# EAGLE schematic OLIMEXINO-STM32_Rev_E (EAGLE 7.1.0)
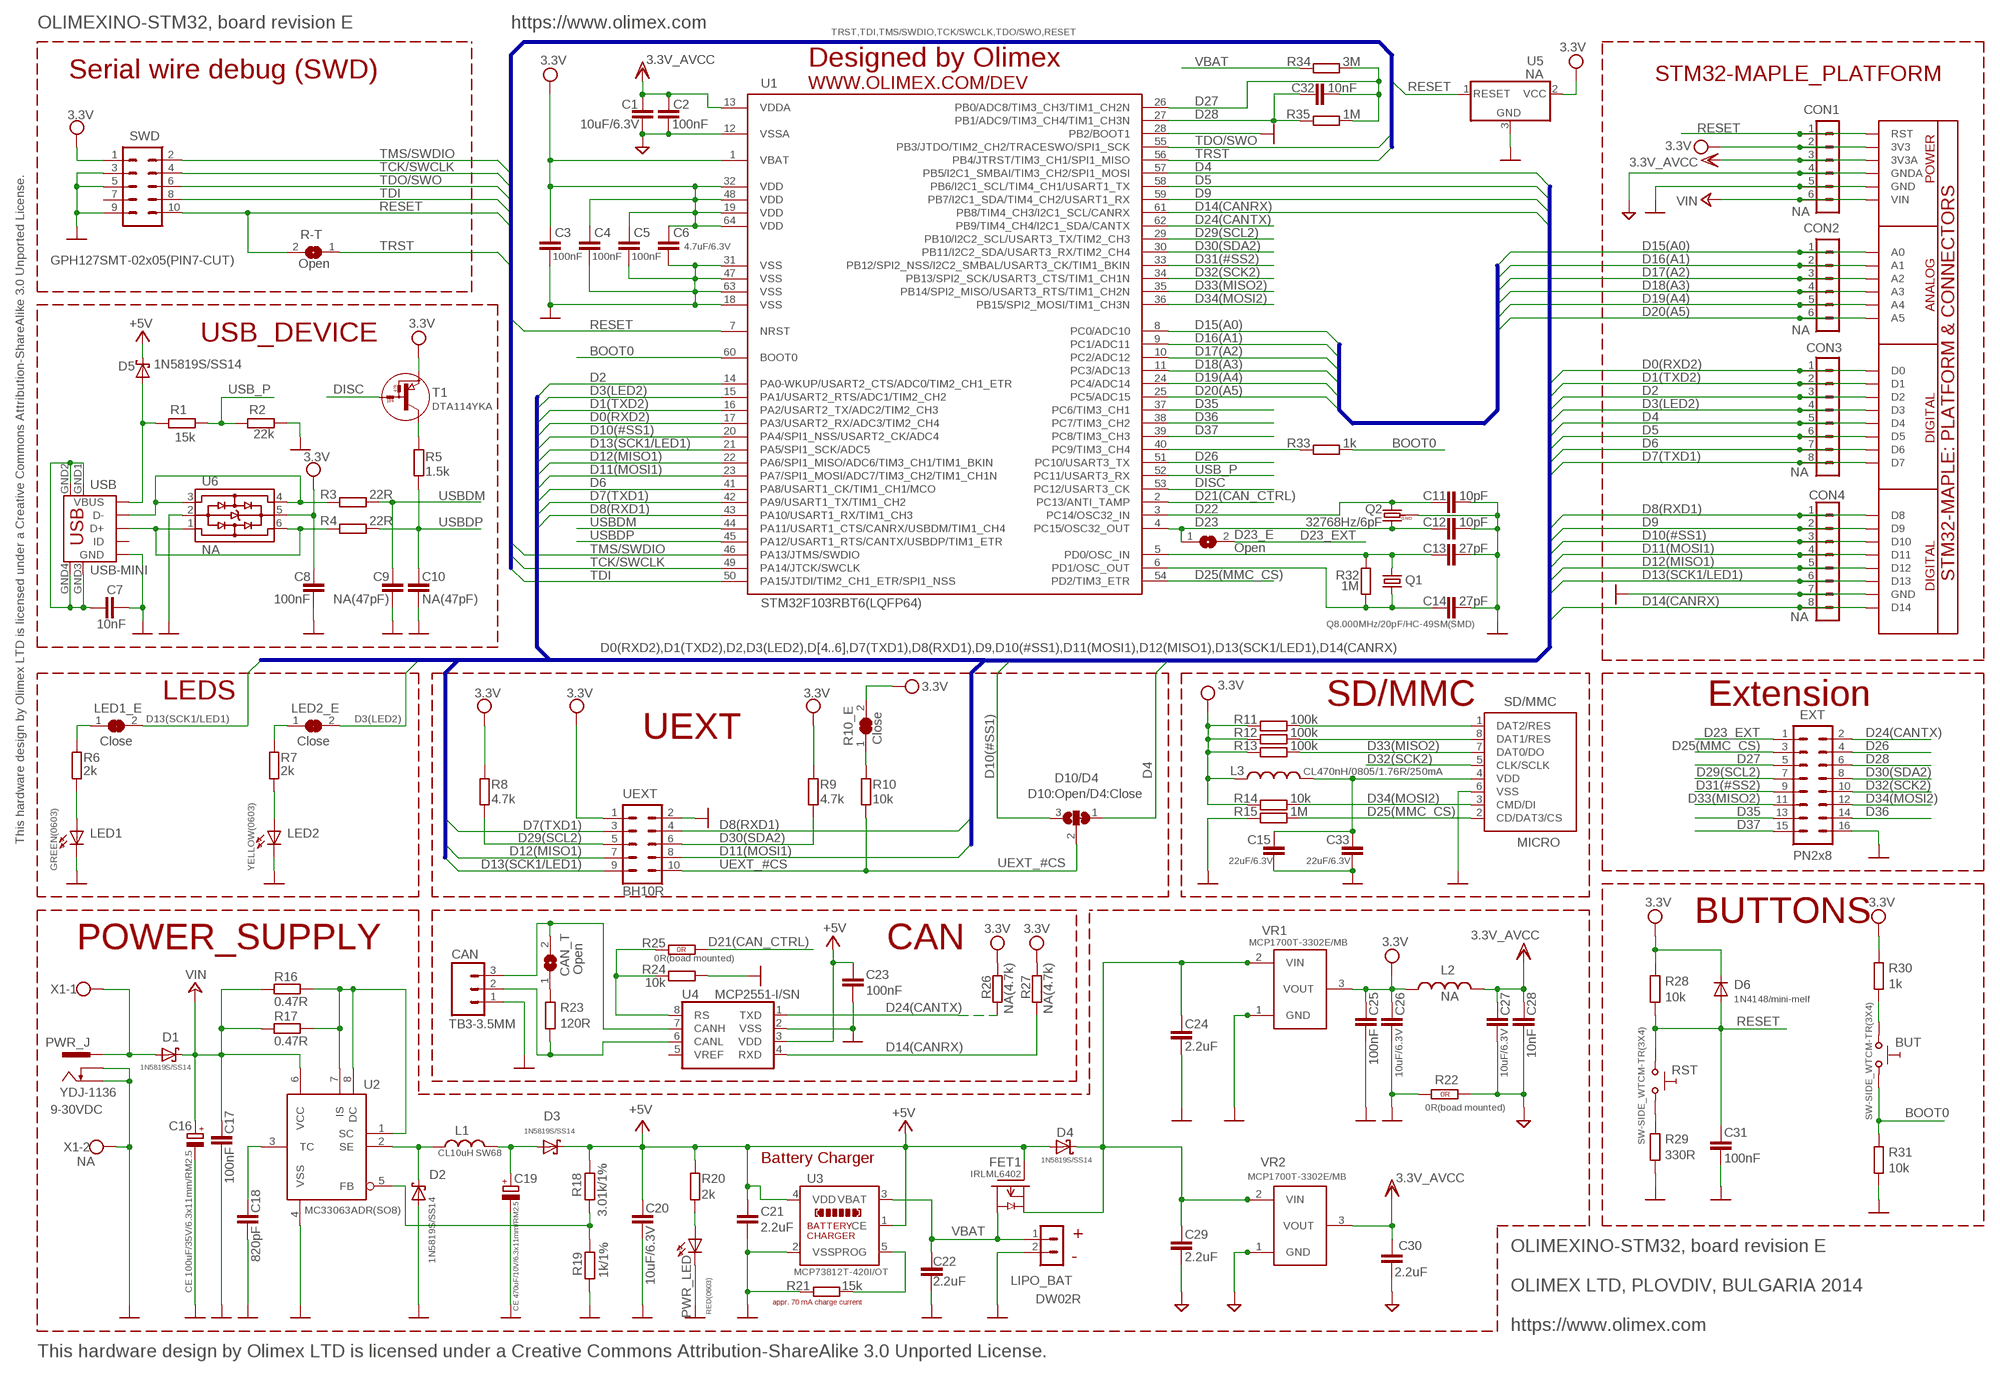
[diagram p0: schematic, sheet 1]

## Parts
BUT  SW-SIDE_WTCM-TR(3X4)  SW-TAKTSIDE_WTCM-TR(3X4)  [SW_TAKT3X4]
C1  10uF/6.3V  C-EUC0805_5MIL_DWS  [C0805_5MIL_DWS]
C2  100nF  C-EUC0603_DWS  [C0603_DWS]
C3  100nF  C-EUC0603_DWS  [C0603_DWS]
C4  100nF  C-EUC0603_DWS  [C0603_DWS]
C5  100nF  C-EUC0603_DWS  [C0603_DWS]
C6  4.7uF/6.3V  C-EUC0603_DWS  [C0603_DWS]
C7  10nF  C-EUC0603_DWS  [C0603_DWS]
C8  100nF  C-EUC0603_DWS  [C0603_DWS]
C9  NA(47pF)  C-EUC0603_DWS_NA  [C0603_DWS_NA]
C10  NA(47pF)  C-EUC0603_DWS_NA  [C0603_DWS_NA]
C11  10pF  C-EUC0603_DWS  [C0603_DWS]
C12  10pF  C-EUC0603_DWS  [C0603_DWS]
C13  27pF  C-EUC0603_DWS  [C0603_DWS]
C14  27pF  C-EUC0603_DWS  [C0603_DWS]
C15  22uF/6.3V  C-EUC0603_DWS  [C0603_DWS]
C16  CE 100uF/35V/6.3x11mm/RM2.5  CPOL-EUE2.5-6.3  [E2,5-6,3]
C17  100nF  C-EUC0603_DWS  [C0603_DWS]
C18  820pF  C-EUC0603_DWS  [C0603_DWS]
C19  CE 470uF/10V/6.3x11mm/RM2.5  CPOL-EUE2.5-6.3  [E2,5-6,3]
C20  10uF/6.3V  C-EUC0805_5MIL_DWS  [C0805_5MIL_DWS]
C21  2.2uF  C-EUC0603_DWS  [C0603_DWS]
C22  2.2uF  C-EUC0603_DWS  [C0603_DWS]
C23  100nF  C-EUC0603_DWS  [C0603_DWS]
C24  2.2uF  C-EUC0603_DWS  [C0603_DWS]
C25  100nF  C-EUC0603_DWS  [C0603_DWS]
C26  10uF/6.3V  C-EUC0805_5MIL_DWS  [C0805_5MIL_DWS]
C27  10uF/6.3V  C-EUC0805_5MIL_DWS  [C0805_5MIL_DWS]
C28  10nF  C-EUC0603_DWS  [C0603_DWS]
C29  2.2uF  C-EUC0603_DWS  [C0603_DWS]
C30  2.2uF  C-EUC0603_DWS  [C0603_DWS]
C31  100nF  C-EUC0603_DWS  [C0603_DWS]
C32  10nF  C-EUC0603_DWS  [C0603_DWS]
C33  22uF/6.3V  C-EUC0603_DWS  [C0603_DWS]
CAN  TB3-3.5MM  CON33.5MM  [CON3/3.5MM]
CAN_T  Open  SJSJ_SMALLER  [SJ_1_SMALLER]
CON1  NA  CON6PN1X6  [PN1X6]
CON2  NA  CON6PN1X6  [PN1X6]
CON3  NA  CON8PN1X8  [PN1X8]
CON4  NA  CON8PN1X8  [PN1X8]
D1  1N5819S/SS14  SCHOTKKY7.62SS2  [MLL-41]
D2  1N5819S/SS14  SCHOTKKY7.62SS2  [MLL-41]
D3  1N5819S/SS14  SCHOTKKY7.62SS2  [MLL-41]
D4  1N5819S/SS14  SCHOTKKY7.62SS2  [MLL-41]
D5  1N5819S/SS14  SCHOTKKY7.62SS2  [MLL-41]
D6  1N4148/mini-melf  DSMD  [MINI-MELF]
D10/D4  D10:Open/D4:Close  SJ2W3  [SJ_2_SMALL]
D23_E  Open  SJSJ_SMALLER  [SJ_1_SMALLER]
EXT  PN2x8  ML16HN2X8  [HN2X8-MALE]
FET1  IRLML6402  [SOT23]
L1  CL10uH SW68  LSW68  [SW68]
L2  NA  L-USL3216C  [L3216C]
L3  CL470nH/0805/1.76R/250mA  L-USL0805_5MIL_DWS  [L0805_5MIL_DWS]
LED1  GREEN(0603)  LED0603DWS  [LED-0603]
LED1_E  Close  SJSJ_1_SMALLER_CLOSE  [SJ_1_SMALLER_CLOSE]
LED2  YELLOW(0603)  LED0603DWS  [LED-0603]
LED2_E  Close  SJSJ_1_SMALLER_CLOSE  [SJ_1_SMALLER_CLOSE]
LIPO_BAT  DW02R  CON2DW02R  [DW02R]
PLATFORM1  STM32-MAPLE_PLATFORM  [STM32-MAPLE_PATFORM]
PWR_J  YDJ-1136  PWR-JAKPWR_JACK_UNI_MILLING  [PWR_JACK_UNI_MILLING]
PWR_LED  RED(0603)  LED0603DWS  [LED-0603]
Q1  Q8.000MHz/20pF/HC-49SM(SMD)  HC49/S1  [HC49/SMD2_THIN]
Q2  32768Hz/6pF  Q_GND1  [TC26H_3_REPAIR_SMD]
R1  15k  R-EU_R0603_5MIL_DWS  [R0603_5MIL_DWS]
R2  22k  R-EU_R0603_5MIL_DWS  [R0603_5MIL_DWS]
R3  22R  R-EU_R0603_5MIL_DWS  [R0603_5MIL_DWS]
R4  22R  R-EU_R0603_5MIL_DWS  [R0603_5MIL_DWS]
R5  1.5k  R-EU_R0603_5MIL_DWS  [R0603_5MIL_DWS]
R6  2k  R-EU_R0603_5MIL_DWS  [R0603_5MIL_DWS]
R7  2k  R-EU_R0603_5MIL_DWS  [R0603_5MIL_DWS]
R8  4.7k  R-EU_R0603_5MIL_DWS  [R0603_5MIL_DWS]
R9  4.7k  R-EU_R0603_5MIL_DWS  [R0603_5MIL_DWS]
R10  10k  R-EU_R0603_5MIL_DWS  [R0603_5MIL_DWS]
R10_E  Close  SJSJ_1_SMALLER_CLOSE  [SJ_1_SMALLER_CLOSE]
R11  100k  R-EU_R0603_5MIL_DWS  [R0603_5MIL_DWS]
R12  100k  R-EU_R0603_5MIL_DWS  [R0603_5MIL_DWS]
R13  100k  R-EU_R0603_5MIL_DWS  [R0603_5MIL_DWS]
R14  10k  R-EU_R0603_5MIL_DWS  [R0603_5MIL_DWS]
R15  1M  R-EU_R0603_5MIL_DWS  [R0603_5MIL_DWS]
R16  0.47R  R-EU_R1206_5MIL_WS  [R1206_5MIL_WS]
R17  0.47R  R-EU_R1206_5MIL_WS  [R1206_5MIL_WS]
R18  3.01k/1%  R-EU_R0603_5MIL_DWS  [R0603_5MIL_DWS]
R19  1k/1%  R-EU_R0603_5MIL_DWS  [R0603_5MIL_DWS]
R20  2k  R-EU_R0603_5MIL_DWS  [R0603_5MIL_DWS]
R21  15k  R-EU_R0603_5MIL_DWS  [R0603_5MIL_DWS]
R22  0R(boad mounted)  R_0R0R(NA)  [0603_0R]
R23  120R  R-EU_R1206_5MIL_WS  [R1206_5MIL_WS]
R24  10k  R-EU_R0603_5MIL_DWS  [R0603_5MIL_DWS]
R25  0R(boad mounted)  R_0R0R(NA)  [0603_0R]
R26  NA(4.7k)  R-EU_R0603_5MIL_DWS_NA  [R0603_5MIL_DWS_NA]
R27  NA(4.7k)  R-EU_R0603_5MIL_DWS_NA  [R0603_5MIL_DWS_NA]
R28  10k  R-EU_R0603_5MIL_DWS  [R0603_5MIL_DWS]
R29  330R  R-EU_R0603_5MIL_DWS  [R0603_5MIL_DWS]
R30  1k  R-EU_R0603_5MIL_DWS  [R0603_5MIL_DWS]
R31  10k  R-EU_R0603_5MIL_DWS  [R0603_5MIL_DWS]
R32  1M  R-EU_R0603_5MIL_DWS  [R0603_5MIL_DWS]
R33  1k  R-EU_R0603_5MIL_DWS  [R0603_5MIL_DWS]
R34  3M  R-EU_R0603_5MIL_DWS  [R0603_5MIL_DWS]
R35  1M  R-EU_R0603_5MIL_DWS  [R0603_5MIL_DWS]
R-T  Open  SJSJ_1_THE_SMALLEST  [SJ_1_THE_SMALLEST]
RST  SW-SIDE_WTCM-TR(3X4)  SW-TAKTSIDE_WTCM-TR(3X4)  [SW_TAKT3X4]
SD/MMC  MICRO  MICRO_SD/MMC  [TFR-MEM-CON]
SWD  GPH127SMT-02x05(PIN7-CUT)  ML10M50  [ML10_50MILS_M]
T1  DTA114YKA  DIGITAL_TRANSISTORS-PNPDTA114YKA  [SOT-23]
U1  STM32F103RBT6(LQFP64)  STM32F103RBT6LQFP64  [LPTQFP64]
U2  MC33063ADR(SO8)  MC34063A2  [SO-8]
U3  MCP73812T-420I/OT  MCP7381XSOT-23-5  [SOT-23-5]
U4  MCP2551-I/SN  [SO-08_THIN]
U5  NA  RESETMCP130T-300-I/TT  [SOT23]
U6  NA  USBLC6-2  [USBLC6-2P6]
UEXT  BH10R  ML10R  [BH10R]
USB  USB-MINI  MINI_USB9  [USB_MINI_9PIN]
VR1  MCP1700T-3302E/MB  MCP1700-REP1  [SOT89_REP_THERMALOFF]
VR2  MCP1700T-3302E/MB  MCP1700-REP1  [SOT89_REP_THERMALOFF]
X1  NA  W237-102  [W237-102]

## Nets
+5V: C20.1 C21.1 C23.1 D3.K(C) D4.A D5.K(C) FET1.1(G) R18.1 R20.1 U3.1(CE) U3.4(VDD) U4.3(VDD)
+5V_USB: D5.A R1.1 USB.VBUS
+24V: C16.+ C17.1 CON1.6 D1.K(C) PLATFORM1.VIN R16.1 R17.1 U2.6(VCC) ; supply symbol labelled VIN
AGND: C1.1 C2.1 C27.2 C28.2 C29.2 C30.2 CON1.4 PLATFORM1.GNDA R22.2(1.2) U1.12(VSSA) VR2.1(GND)
BOOT0: BUT.2_1 R31.1 R33.1 U1.60(BOOT0)
D0(RXD2): CON3.1 PLATFORM1.D0 U1.17(PA3/USART2_RX/ADC3/TIM2_CH4)
D1(TXD2): CON3.2 PLATFORM1.D1 U1.16(PA2/USART2_TX/ADC2/TIM2_CH3)
D2: CON3.3 PLATFORM1.D2 U1.14(PA0-WKUP/USART2_CTS/ADC0/TIM2_CH1_ETR)
D3(LED2): CON3.4 LED2_E.2 PLATFORM1.D3 U1.15(PA1/USART2_RTS/ADC1/TIM2_CH2)
D4: CON3.5 D10/D4.1 PLATFORM1.D4 U1.57(PB5/I2C1_SMBAI/TIM3_CH2/SPI1_MOSI)
D5: CON3.6 PLATFORM1.D5 U1.58(PB6/I2C1_SCL/TIM4_CH1/USART1_TX)
D6: CON3.7 PLATFORM1.D6 U1.41(PA8/USART1_CK/TIM1_CH1/MCO)
D7(TXD1): CON3.8 PLATFORM1.D7 U1.42(PA9/USART1_TX/TIM1_CH2) UEXT.3
D8(RXD1): CON4.1 PLATFORM1.D8 U1.43(PA10/USART1_RX/TIM1_CH3) UEXT.4
D9: CON4.2 PLATFORM1.D9 U1.59(PB7/I2C1_SDA/TIM4_CH2/USART1_RX)
D10(#SS1): CON4.3 D10/D4.3 PLATFORM1.D10 U1.20(PA4/SPI1_NSS/USART2_CK/ADC4)
D11(MOSI1): CON4.4 PLATFORM1.D11 U1.23(PA7/SPI1_MOSI/ADC7/TIM3_CH2/TIM1_CH1N) UEXT.8
D12(MISO1): CON4.5 PLATFORM1.D12 U1.22(PA6/SPI1_MISO/ADC6/TIM3_CH1/TIM1_BKIN) UEXT.7
D13(SCK1/LED1): CON4.6 LED1_E.2 PLATFORM1.D13 U1.21(PA5/SPI1_SCK/ADC5) UEXT.9
D14(CANRX): CON4.8 PLATFORM1.D14 R27.2 U1.61(PB8/TIM4_CH3/I2C1_SCL/CANRX) U4.4(RXD)
D15(A0): CON2.1 PLATFORM1.A0 U1.8(PC0/ADC10)
D16(A1): CON2.2 PLATFORM1.A1 U1.9(PC1/ADC11)
D17(A2): CON2.3 PLATFORM1.A2 U1.10(PC2/ADC12)
D18(A3): CON2.4 PLATFORM1.A3 U1.11(PC3/ADC13)
D19(A4): CON2.5 PLATFORM1.A4 U1.24(PC4/ADC14)
D20(A5): CON2.6 PLATFORM1.A5 U1.25(PC5/ADC15)
D21(CAN_CTRL): R25.1(1.1) U1.2(PC13/ANTI_TAMP)
D22: C11.1 Q2.2 U1.3(PC14/OSC32_IN)
D23: C12.1 D23_E.1 Q2.1 U1.4(PC15/OSC32_OUT)
D23_EXT: D23_E.2 EXT.1
D24(CANTX): EXT.2 R26.2 U1.62(PB9/TIM4_CH4/I2C1_SDA/CANTX) U4.1(TXD)
D25(MMC_CS): EXT.3 R15.2 SD/MMC.2(CD/DAT3/CS) U1.54(PD2/TIM3_ETR)
D26: EXT.4 U1.51(PC10/USART3_TX)
D27: C32.2 EXT.5 R34.1 R35.1 U1.26(PB0/ADC8/TIM3_CH3/TIM1_CH2N)
D28: C32.1 EXT.6 R35.2 U1.27(PB1/ADC9/TIM3_CH4/TIM1_CH3N)
D29(SCL2): EXT.7 R8.1 U1.29(PB10/I2C2_SCL/USART3_TX/TIM2_CH3) UEXT.5
D30(SDA2): EXT.8 R9.1 U1.30(PB11/I2C2_SDA/USART3_RX/TIM2_CH4) UEXT.6
D31(#SS2): EXT.9 U1.33(PB12/SPI2_NSS/I2C2_SMBAL/USART3_CK/TIM1_BKIN)
D32(SCK2): EXT.10 SD/MMC.5(CLK/SCLK) U1.34(PB13/SPI2_SCK/USART3_CTS/TIM1_CH1N)
D33(MISO2): EXT.11 R13.2 SD/MMC.7(DAT0/DO) U1.35(PB14/SPI2_MISO/USART3_RTS/TIM1_CH2N)
D34(MOSI2): EXT.12 R14.2 SD/MMC.3(CMD/DI) U1.36(PB15/SPI2_MOSI/TIM1_CH3N)
D35: EXT.13 U1.37(PC6/TIM3_CH1)
D36: EXT.14 U1.38(PC7/TIM3_CH2)
D37: EXT.15 U1.39(PC8/TIM3_CH3)
D+: R4.2 U6.1 U6.6 USB.D+
D-: R3.2 U6.3 U6.4 USB.D-
DISC: T1.1(B) U1.53(PC12/USART3_CK)
GND [pwr]: C3.1 C4.1 C5.1 C6.1 C7.2 C8.1 C9.2 C10.2 C11.2 C12.2 C13.2 C14.2 C15.2 C16.- C17.2 C18.2 C19.- C20.2 C21.2 C22.2 C23.2 C24.2 C25.2 C26.2 C31.2 C33.2 CAN.1 CON1.5 CON4.7 D2.A EXT.16 LED1.C LED2.C LIPO_BAT.2 PLATFORM1.GND PLATFORM1.GND@1(GND) PWR_J.- PWR_J.-- PWR_LED.C Q2.GND R2.2 R15.1 R19.2 R21.1 R22.1(1.1) R24.1 R29.1 R31.2 SD/MMC.6(VSS) SWD.3 SWD.5 SWD.9 U1.18(VSS) U1.28(PB2/BOOT1) U1.31(VSS) U1.47(VSS) U1.63(VSS) U2.4(VSS) U3.2(VSS) U4.2(VSS) U5.3(GND) U6.2 UEXT.2 USB.GND VR1.1(GND) X1.2
MCIDAT1: R12.2 SD/MMC.8(DAT1/RES)
MCIDAT2: R11.2 SD/MMC.1(DAT2/RES)
MMC_PWR: C15.1 C33.1 L3.2 SD/MMC.4(VDD)
N$1: CAN_T.1 R23.2
N$2: LED1_E.1 R6.2
N$3: R24.2 R25.2(1.2) U4.8(RS)
N$4: R10.2 R10_E.1
N$5: LED2.A R7.1
N$6: LED2_E.1 R7.2
N$7: C19.+ D3.A L1.2
N$8: PWR_LED.A R20.2
N$11 [pwr]: R29.2 RST.1_1
N$12 [pwr]: BUT.1_1 R30.2
N$13: D1.A PWR_J.+ X1.1
N$22: R21.2 U3.5(PROG)
N$23: LED1.A R6.1
N$33: C18.1 U2.3(TC)
N$34: C24.1 C29.1 D4.K(C) FET1.2(S) VR1.2(VIN) VR1.P$2(VIN1) VR2.2(VIN) VR2.P$2(VIN1)
N$41: C13.1 Q1.2 R32.2 U1.5(PD0/OSC_IN)
N$42: C14.1 Q1.1 R32.1 U1.6(PD1/OSC_OUT)
N$56: R5.2 T1.3(C)
N$61: R18.2 R19.1 U2.5(FB)
N$64: R16.2 R17.2 U2.1(SC) U2.7(IS) U2.8(DC)
N$67 [pwr]: D2.K(C) L1.1 U2.2(SE)
N$76: CAN.2 R23.1 U4.6(CANL)
N$77: CAN.3 CAN_T.2 U4.7(CANH)
N$82: R33.2 U1.40(PC9/TIM3_CH4)
RESET: C31.1 CON1.1 D6.A PLATFORM1.RST R28.2 R-T.2 RST.2_1 SWD.10 U1.7(NRST) U5.1(RESET)
TCK/SWCLK: SWD.4 U1.49(PA14/JTCK/SWCLK)
TDI: SWD.8 U1.50(PA15/JTDI/TIM2_CH1_ETR/SPI1_NSS)
TDO/SWO: SWD.6 U1.55(PB3/JTDO/TIM2_CH2/TRACESWO/SPI1_SCK)
TMS/SWDIO: SWD.2 U1.46(PA13/JTMS/SWDIO)
TRST: R-T.1 U1.56(PB4/JTRST/TIM3_CH1/SPI1_MISO)
UEXT_#CS: D10/D4.2 R10.1 UEXT.10
USB_P: R1.2 R2.1 U1.52(PC11/USART3_RX)
USB_SHIELD: C7.1 USB.GND1 USB.GND2 USB.GND3 USB.GND4
USBDM: C9.1 R3.1 U1.44(PA11/USART1_CTS/CANRX/USBDM/TIM1_CH4)
USBDP: C10.1 R4.1 R5.1 U1.45(PA12/USART1_RTS/CANTX/USBDP/TIM1_ETR)
VBAT: C22.1 FET1.3(D) LIPO_BAT.1 R34.2 U3.3(VBAT)
VCC: C3.2 C4.2 C5.2 C6.2 C8.2 C25.1 C26.1 CON1.2 D6.C(K) L2.1 L3.1 PLATFORM1.3V3 R8.2 R9.2 R10_E.2 R11.1 R12.1 R13.1 R14.1 R26.1 R27.1 R28.1 R30.1 SWD.1 T1.2(E) U1.1(VBAT) U1.19(VDD) U1.32(VDD) U1.48(VDD) U1.64(VDD) U5.2(VCC) U6.5 UEXT.1 VR1.3(VOUT) ; supply symbol labelled 3.3V
VDD: C1.2 C2.2 C27.1 C28.1 C30.1 CON1.3 L2.2 PLATFORM1.3V3A U1.13(VDDA) VR2.3(VOUT) ; supply symbol labelled 3.3V_AVCC
Unconnected: SWD.7 U4.5(VREF) USB.ID

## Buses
D15(A0),D16(A1),D17(A2),D18(A3),D19(A4),D20(A5)
D0(RXD2),D1(TXD2),D2,D3(LED2),D[4..6],D7(TXD1),D8(RXD1),D9,D10(#SS1),D11(MOSI1),D12(MISO1),D13(SCK1/LED1),D14(CANRX)
TRST,TDI,TMS/SWDIO,TCK/SWCLK,TDO/SWO,RESET

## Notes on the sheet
- OLIMEXINO-STM32, board revision E | https://www.olimex.com
- Designed by Olimex
- Serial wire debug (SWD) | STM32-MAPLE_PLATFORM
- WWW.OLIMEX.COM/DEV
- USB_DEVICE
- LEDS | SD/MMC | Extension
- UEXT
- This hardware design by Olimex LTD is licensed under a Creative Commons Attribution-ShareAlike 3.0 Unported License.
- BUTTONS
- POWER_SUPPLY | CAN
- 9-30VDC
- Battery Charger
- +
- - | OLIMEXINO-STM32, board revision E
- OLIMEX LTD, PLOVDIV, BULGARIA 2014
- appr. 70 mA charge current
- https://www.olimex.com
- This hardware design by Olimex LTD is licensed under a Creative Commons Attribution-ShareAlike 3.0 Unported License.

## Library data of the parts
BUT RST = gogo:SW-TAKT
C1-C15 C17 C18 C20-C33 = rcl:C-EU: CAPACITOR, European symbol
C16 C19 = rcl:CPOL-EU: POLARIZED CAPACITOR, European symbol
CAN = DOUBLE-SIDE:CON3: CONNECTORS - 3 PINS
CAN_T D23_E LED1_E LED2_E R10_E R-T = jumper:SJ: SMD solder JUMPER
CON1 CON2 = Penko:CON6: CONNECTORS - 6 PINS
CON3 CON4 = Penko:CON8
D1-D5 = gogo:SCHOTKKY7.62SS
D6 = DOUBLE-SIDE:D: DIODES
D10/D4 = jumper:SJ2W: SMD solder JUMPER
EXT = con-harting-ml:ML16: HARTING
FET1 = gogo:IRLML6402
L1 = DOUBLE-SIDE:L
L2 L3 = rcl:L-US: INDUCTOR, American symbol
LED1 LED2 PWR_LED = DOUBLE-SIDE:LED
LIPO_BAT = Penko:CON2
PLATFORM1 = OLIMEX_CASES:STM32-MAPLE_PLATFORM
PWR_J = gogo:PWR-JAK
Q1 = crystal:HC49/S: CRYSTAL
Q2 = crystal:Q_GND
R1-R21 R23 R24 R26-R35 = rcl:R-EU_: RESISTOR, European symbol
R22 R25 = OLIMEX_DISCRET:R_0R
SD/MMC = OLIMEX_CONNECTORS:MICRO_SD/MMC
SWD UEXT = con-harting-ml:ML10: HARTING
T1 = OLIMEX_DISCRET:DIGITAL_TRANSISTORS-PNP: DTA114YKA Digital Transistor - PNP
U1 = OLIMEX_IC:STM32F103RBT6: STM32F103 - Advanced ARM-based 32-bit MCU with Flash, USB, CAN, 8 16-bit timers, 2 ADC, 2 DAC, 11 communication interfaces
U2 = MPLAB_ICD2:MC34063A
U3 = OLIMEX_DISCRET:MCP7381X
U4 = arm:MCP2551
U5 = gogo:RESET: Microcontroller Supervisory Circuit with Open Drain Output
U6 = OLIMEX_IC:USBLC6-2
USB = OLIMEX_CONNECTORS:MINI_USB9
VR1 VR2 = OLIMEX_DISCRET:MCP1700-REP
X1 = con-wago-500:W237-102: WAGO SCREW CLAMP

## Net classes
0 default: width 0.241 mm, drill 0.584 mm, clearance 0.241 mm
1 pwr: width 0.25 mm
